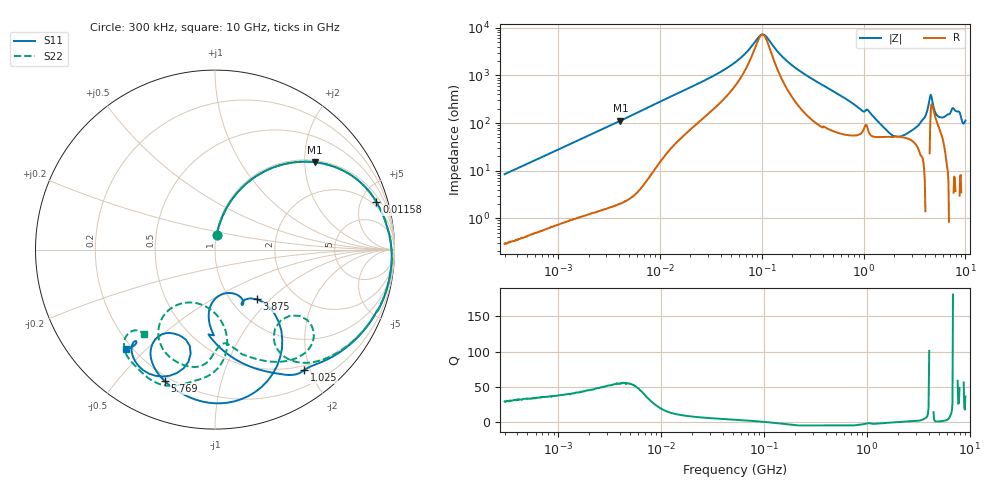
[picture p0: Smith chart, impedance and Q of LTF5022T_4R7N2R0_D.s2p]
! S-Parameter Data Generated by TDK Corporation
! Copyright(C) 2020 TDK Corporation.
! All Rights Reserved.
! TDK P/N: LTF5022T-4R7N2R0-D (Inductor)
! Property: L=4.7uH at 100kHz
! Size(LxWxT): 6.5x5x2.2mm
! Model Type: s2p (Touchstone File Format Version 1.0)
! Frequency: DC=Yes Start=0.3MHz Stop=10000MHz 802points Log-sweep
! Model Generated on Apr. 23, 2020
! Port Assignments:
!  1 ---@@@--- 2
! Applicable Conditions:
!  Temperature = 25 degC
!  DC Bias Current = 0 A
!  Small Signal Operation
! Terms and conditions regarding TDK Simulation Models
! (1)This simulation model is being provided solely for informational purposes. Please refer to the specifications of the products in terms of detailed characteristics of such products.
! (2)In no event shall TDK Corporation of any of its subsidiaries be liable for any loss or damage arising, directly or indirectly,
!  From any information contained in this simulation model, including, but not limited to loss or damages arising from any inaccuracies, omissions or errors in connection with such information.
! (3)Any and all copyrights on this simulation model are owned by TDK Corporation.
!  Duplication or redistribution of this simulation model without prior written permission from TDK Corporation is prohibited.
! (4)This simulation model is subject to any modification or change without any prior notice.
! (5)Neither TDK Corporation nor any of its subsidiaries shall make any warranty, express or implied,
!  Including but not limited to the correctness, implied warranties of merchantability and fitness for a particular purpose with respect to this simulation models.
! (6)The use of this simulation model shall be deemed to have consented to the terms and conditions hereof.
# Hz S MA R 50
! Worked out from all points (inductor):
!   801 points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, 300 kHz to 10 GHz, reference 50 ohm
!   read as one part in series: L = 4.44 uH near 318.3 kHz
!   highest Q = 55.1 at 4.116 MHz (marker M1), where L = 4.33 uH
!   self-resonance near 101.6 MHz
!   S11 on the Smith chart (normalised r, x): 300 kHz: 1.01, +0.17; 11.58 MHz: 1.51, +6.61; 1.025 GHz: 0.43, -1.91; 3.875 GHz: 1.31, -0.83; 5.769 GHz: 0.18, -0.67; 10 GHz: 0.18, -0.43
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300000  0.0837 83.4  0.9936 -4.8  0.9937 -4.8  0.08373 83.1
1713600  0.4192 63.8  0.8981 -24.8  0.8982 -24.8  0.4192 63.8
4115543  0.7387 41.2  0.6608 -47.7  0.6609 -47.7  0.7386 41.2
9671944  0.9229 19.7  0.3418 -67.5  0.3419 -67.5  0.9229 19.7
1.158341e7  0.9377 16.4  0.2887 -69.6  0.2888 -69.6  0.9376 16.4
5.477226e7  0.9819 1.2  0.05251 -70.1  0.05251 -70.1  0.9819 1.2
1.038383e8  0.9864 -3.3  0.01363 4.0  0.01362 4.1  0.9864 -3.2
3.126428e8  0.9774 -16.0  0.1138 66.3  0.1138 66.3  0.9777 -15.7
8.758105e8  0.8648 -46.2  0.3342 29.6  0.3341 29.6  0.8335 -48.7
1.024756e9  0.836 -53.4  0.3275 15.3  0.3277 15.4  0.5854 -56.1
1.180962e9  0.7733 -63.3  0.3921 19.7  0.3923 19.6  0.7555 -44.7
1.767019e9  0.5474 -87.0  0.5156 -20.5  0.5153 -20.5  0.6384 -70.9
2.882439e9  0.2706 -89.0  0.5087 -80.3  0.5081 -80.3  0.5275 -85.7
3.874538e9  0.3626 -49.7  0.2877 -135.5  0.2873 -135.4  0.6671 -104.3
4.22443e9  0.6272 -53.3  0.182 -154.2  0.1811 -154.2  0.6261 -117.6
4.574322e9  0.8085 -71.3  0.07597 -123.3  0.0753 -122.3  0.5013 -127.2
5.157474e9  0.8466 -96.0  0.1948 -100.3  0.1961 -99.9  0.3154 -108.8
5.76861e9  0.7837 -111.0  0.2333 -130.9  0.2347 -130.8  0.4358 -83.1
6.737565e9  0.5547 -121.9  0.1676 -158.4  0.167 -158.5  0.7114 -94.0
7.316673e9  0.5277 -107.8  0.1421 -174.2  0.142 -173.8  0.7813 -104.8
8.658336e9  0.7658 -125.4  0.0937 170.9  0.09283 170.6  0.7668 -130.0
1e10  0.7401 -131.9  0.124 139.7  0.1242 141.2  0.6165 -130.0
